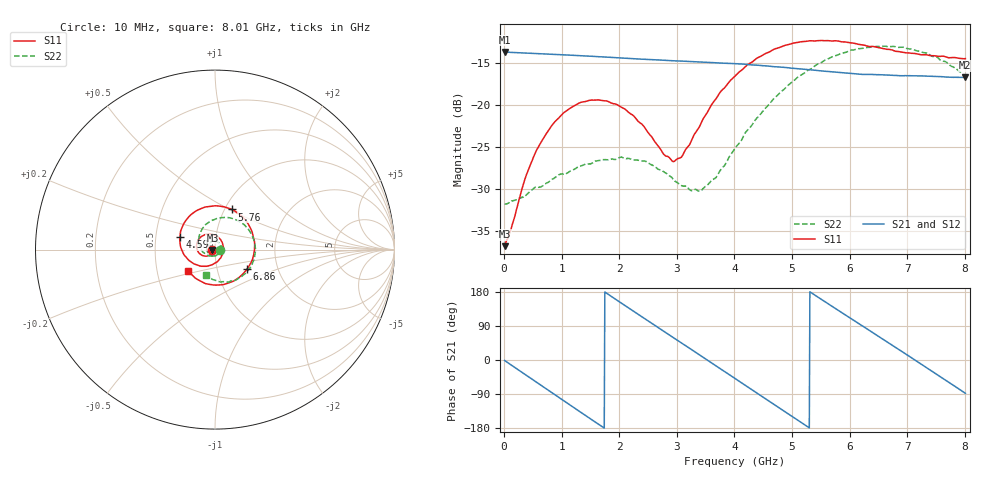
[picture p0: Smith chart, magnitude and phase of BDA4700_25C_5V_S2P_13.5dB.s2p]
!Agilent Technologies,E5071B,MY42404982,A.09.10
!Date: Mon Oct 20 13:32:55 2025
!Data & Calibration Information:
!Freq	S11:SOLT2(ON)	S21:SOLT2(ON)	S12:SOLT2(ON)	S22:SOLT2(ON)
# Hz S RI R 50
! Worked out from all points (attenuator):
!   801 points, 10 MHz to 8.01 GHz, reference 50 ohm
!   highest |S21| = -13.61 dB at 10 MHz (marker M1); lowest = -16.7 dB at 8 GHz (marker M2)
!   lowest |S11| = -36.9 dB at 10 MHz (marker M3), VSWR 1.03, Z = 48.6 - j0.141 ohm
!   |S11| at or under -10 dB: start of sweep to end of sweep
!   |S22| runs from -31.8 to -12.9 dB; largest |S21 - S12| = 0.0016
!   S11 on the Smith chart (normalised r, x): 10 MHz: 0.97, -0.00; 4.59 GHz: 0.67, +0.10; 5.76 GHz: 1.08, +0.51; 6.86 GHz: 1.40, -0.31; 8.01 GHz: 0.72, -0.18
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1e7  -0.0143 -0.00146  0.2087 -0.00457  0.2086 -0.00469  0.0258 -0.00097
3.8e8  -0.0261 -0.0271  0.1575 -0.1318  0.1573 -0.1319  0.0208 -0.0201
5.9e8  -0.0429 -0.0361  0.0967 -0.1793  0.0966 -0.1794  0.0125 -0.0299
1e9  -0.0844 -0.0235  -0.0481 -0.1946  -0.0482 -0.1949  -0.0183 -0.0343
1.35e9  -0.1034 0.015  -0.151 -0.1277  -0.1511 -0.1277  -0.0411 -0.0144
1.71e9  -0.0866 0.0621  -0.1944 -0.0116  -0.1945 -0.0114  -0.0441 0.017
2.07e9  -0.0401 0.0873  -0.1602 0.1049  -0.1603 0.105  -0.0242 0.042
2.68e9  0.0397 0.0408  0.0155 0.1861  0.0156 0.186  0.0254 0.0326
2.97e9  0.0456 -0.0102  0.1029 0.153  0.1029 0.1527  0.0336 0.0102
3.4e9  -0.000631 -0.0752  0.1771 0.0402  0.1773 0.0402  0.0178 -0.0249
3.69e9  -0.0604 -0.0927  0.1721 -0.0506  0.1723 -0.0511  -0.00966 -0.0362
4.01e9  -0.1324 -0.0694  0.1169 -0.1335  0.117 -0.1333  -0.0466 -0.0297
4.59e9  -0.1954 0.0695  -0.052 -0.1635  -0.0518 -0.1637  -0.09 0.0443
4.99e9  -0.1468 0.1818  -0.1412 -0.0886  -0.1416 -0.0889  -0.0696 0.1179
5.35e9  -0.0454 0.2385  -0.1622 0.0115  -0.1623 0.0111  -0.00602 0.1663
5.76e9  0.0947 0.2238  -0.1119 0.1112  -0.1119 0.1114  0.0964 0.1735
6.23e9  0.2041 0.1049  0.00219 0.1529  0.00355 0.153  0.1973 0.0954
6.68e9  0.2096 -0.0514  0.1077 0.1065  0.1079 0.1064  0.2222 -0.0271
6.86e9  0.1795 -0.1075  0.134 0.0683  0.1343 0.0676  0.2079 -0.0777
7.43e9  0.0126 -0.1974  0.1296 -0.0738  0.1295 -0.0743  0.0913 -0.1742
8e9  -0.1481 -0.1193  0.00805 -0.1465  0.00797 -0.1467  -0.0478 -0.1417
8.01e9  -0.1499 -0.1169  0.00543 -0.1467  0.00559 -0.1468  -0.0499 -0.1398
